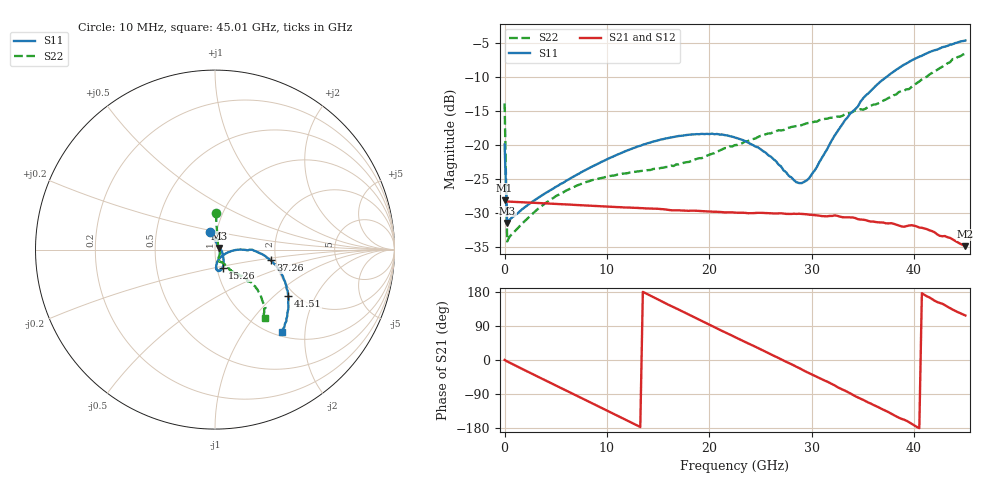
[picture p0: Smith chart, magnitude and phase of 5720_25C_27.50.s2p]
! Device:  ADRF5720
! Description: 0.5dB LSB GaAs MMIC 6-bit Digital Attenuator
! Frequency:  0.000009 -  40 GHz
! Ports:
!	RF1	= Port 1
!	RF2	= Port 2
! Vdd:  3.3 Volt
! Vss:  -3.3 Volt
! Control:  0/3.3 Volt
! State:  27.50 dB attenuation
! Data:  The device was measured using G-S-G Probes on a matrix board.
!  Data was collected using an calibrated 4 port network analyzer.
!  The reference plane for this measurement is at the launchers.
! Note:  Analog Devices supplies this data as a sample of measured data
!  for this product.  Your particular data for this product may vary.
!  Data was taken at 25 degrees C.
!  Analog Devices reserves the right to change this data at anytime.
# GHZ S DB R 45.0
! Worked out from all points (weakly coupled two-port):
!   181 points, 10 MHz to 45.01 GHz, reference 45 ohm
!   highest |S21| = -28.11 dB at 10 MHz (marker M1); lowest = -34.9 dB at 45.01 GHz (marker M2)
!   lowest |S11| = -31.5 dB at 260 MHz (marker M3), VSWR 1.05, Z = 47.3 + j0.872 ohm
!   |S11| at or under -10 dB: start of sweep to 37.28 GHz
!   |S22| runs from -34.2 to -6.5 dB; largest |S21 - S12| = 0.0001
!   S11 on the Smith chart (normalised r, x): 10 MHz: 0.93, +0.18; 15.26 GHz: 1.07, -0.22; 37.26 GHz: 1.88, -0.25; 41.51 GHz: 1.83, -1.24; 45.01 GHz: 1.08, -1.51
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0.01  -19.91 106.4  -28.11 0.2  -28.11 0.1  -13.86 88.8
0.26  -31.47 20.2  -28.30 -3.7  -28.31 -3.7  -34.17 25.0
1.26  -30.07 1.8  -28.37 -17.3  -28.38 -17.3  -32.25 -7.3
3.51  -27.54 -19.4  -28.53 -47.4  -28.53 -47.4  -29.10 -41.1
5.01  -26.15 -30.2  -28.65 -67.2  -28.65 -67.2  -27.51 -55.2
7.76  -23.78 -44.1  -28.87 -103.6  -28.86 -103.6  -25.55 -69.9
12.01  -20.77 -58.5  -29.18 -160.0  -29.18 -160.0  -24.13 -76.4
15.26  -19.18 -67.1  -29.41 156.0  -29.41 156.0  -23.37 -72.5
20.26  -18.31 -79.6  -29.79 89.7  -29.79 89.7  -21.28 -60.1
22.76  -19.00 -85.5  -29.95 57.2  -29.95 57.2  -19.97 -56.2
25.51  -21.11 -84.9  -30.00 21.4  -30.00 21.4  -18.40 -54.8
28.51  -25.47 -58.0  -30.12 -18.0  -30.12 -17.9  -17.20 -54.1
29.51  -25.20 -35.2  -30.18 -31.6  -30.19 -31.6  -16.79 -52.8
30.26  -23.79 -18.5  -30.30 -41.2  -30.30 -41.2  -16.55 -52.9
33.26  -16.32 -0.1  -30.63 -81.0  -30.62 -80.9  -15.43 -49.4
35.26  -12.72 -2.8  -31.03 -108.6  -31.02 -108.6  -14.64 -47.0
37.26  -10.02 -10.9  -31.51 -134.7  -31.50 -134.8  -13.27 -43.8
37.76  -9.44 -13.3  -31.49 -141.3  -31.49 -141.3  -12.95 -43.2
39.51  -7.76 -22.0  -31.83 -164.1  -31.83 -163.9  -11.75 -43.5
41.51  -6.31 -32.4  -32.54 164.9  -32.52 164.7  -9.60 -43.6
43.76  -5.15 -43.9  -33.87 133.0  -33.89 133.1  -7.34 -49.1
45.01  -4.60 -50.8  -34.87 117.5  -34.88 117.4  -6.53 -53.8
